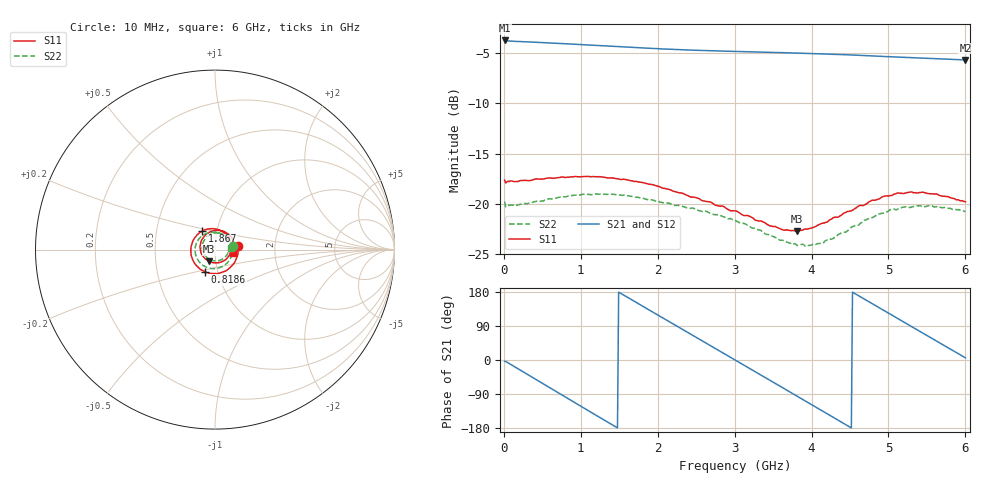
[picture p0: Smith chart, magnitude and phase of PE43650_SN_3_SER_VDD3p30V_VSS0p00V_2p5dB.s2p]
!Keysight Technologies,N5245B,MY57181451,A.13.50.07
!Date: Tuesday, May 07, 2019 07:59:49
!Correction: S11(Full 2 Port(1,2))
!S21(Full 2 Port(1,2))
!S12(Full 2 Port(1,2))
!S22(Full 2 Port(1,2))
!S2P File: Measurements: S11, S21, S12, S22:
# Hz S  dB  R 50
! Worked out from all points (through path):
!   401 points, 10 MHz to 6 GHz, reference 50 ohm
!   highest |S21| = -3.74 dB at 10 MHz (marker M1); lowest = -5.7 dB at 6 GHz (marker M2)
!   group delay of S21, straight-line fit = 330 ps
!   lowest |S11| = -22.8 dB at 3.814 GHz (marker M3), VSWR 1.16, Z = 46.6 - j6.15 ohm
!   |S11| at or under -10 dB: start of sweep to end of sweep
!   |S22| runs from -24.2 to -19.0 dB; largest |S21 - S12| = 0.0053
!   S11 on the Smith chart (normalised r, x): 10 MHz: 1.30, +0.05; 818.6 MHz: 0.87, -0.22; 1.867 GHz: 0.85, +0.18; 6 GHz: 1.22, -0.05
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1e7  -17.65 8.0  -3.74 -3.4  -3.81 -3.3  -19.79 12.5
2.1965e8  -17.69 -32.2  -3.86 -27.5  -3.90 -27.5  -20.06 -32.1
4.5925e8  -17.55 -65.7  -3.94 -56.7  -3.99 -56.7  -19.76 -66.0
8.1865e8  -17.37 -113.5  -4.07 -100.2  -4.12 -100.2  -19.27 -113.5
1.013325e9  -17.31 -138.4  -4.16 -123.6  -4.21 -123.6  -19.08 -137.4
1.4476e9  -17.49 171.0  -4.34 -175.5  -4.40 -175.5  -19.09 174.6
1.8669e9  -18.02 125.7  -4.51 134.7  -4.57 134.7  -19.59 132.8
2.01665e9  -18.29 110.5  -4.57 116.9  -4.62 116.9  -19.78 118.7
2.241275e9  -18.84 87.4  -4.64 90.4  -4.70 90.4  -20.17 97.8
2.4659e9  -19.35 63.7  -4.71 63.9  -4.77 63.9  -20.47 76.4
2.750425e9  -20.15 33.7  -4.78 30.3  -4.83 30.3  -21.08 48.1
3.005e9  -20.71 3.1  -4.83 0.2  -4.89 0.3  -21.64 20.5
3.45425e9  -22.19 -57.9  -4.93 -53.0  -4.97 -52.9  -23.12 -38.2
3.81365e9  -22.76 -115.5  -5.00 -95.6  -5.05 -95.6  -24.16 -94.3
4.008325e9  -22.39 -147.2  -5.04 -118.7  -5.09 -118.7  -24.08 -127.4
4.2629e9  -21.52 173.1  -5.11 -149.0  -5.16 -148.9  -23.53 -169.2
4.5025e9  -20.73 139.1  -5.18 -177.5  -5.24 -177.3  -22.46 154.1
4.7421e9  -19.83 107.9  -5.27 154.1  -5.32 154.3  -21.50 123.1
5.01165e9  -19.21 76.9  -5.36 122.3  -5.41 122.4  -20.65 90.8
5.4609e9  -18.88 31.3  -5.51 69.3  -5.56 69.4  -20.28 46.2
5.745425e9  -19.29 7.0  -5.60 35.7  -5.65 35.8  -20.38 22.0
6e9  -19.80 -11.9  -5.68 5.8  -5.73 5.9  -20.78 4.1
